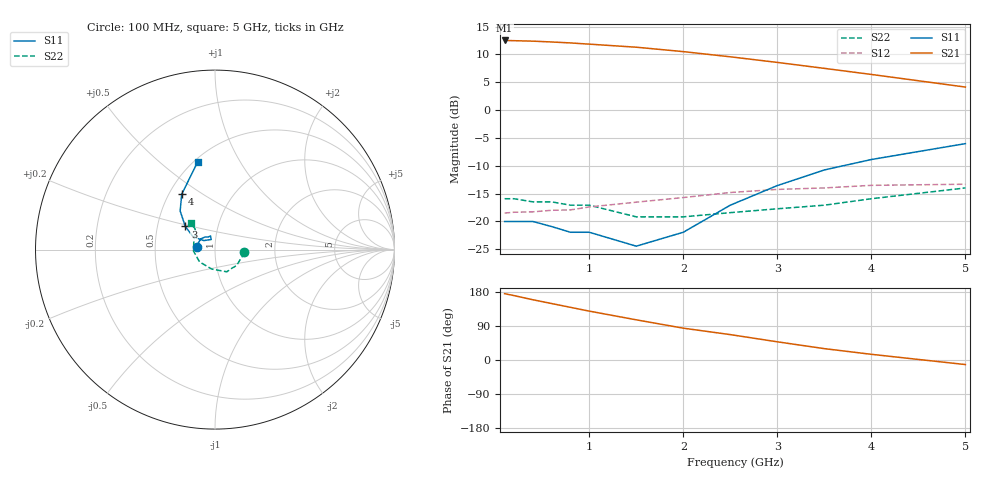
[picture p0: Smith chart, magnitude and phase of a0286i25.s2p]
!  MSA-0286 S AND NOISE PARAMETERS
!  Id=25mA  LAST UPDATED 07-22-92
# ghz s ma r 50
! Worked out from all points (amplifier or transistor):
!   13 points, 100 MHz to 5 GHz, reference 50 ohm
!   highest |S21| = 12.5 dB at 100 MHz (marker M1)
!   |S21| within 3 dB of that: start of sweep to 2.532 GHz
!   unconditionally stable (mu >= 1): start of sweep to end of sweep
!   at 400 MHz: K = 1.20, MAG = 12.6 dB, |S12| = -18.3 dB
!   at 1.5 GHz: K = 1.18, MAG = 11.4 dB, |S12| = -16.5 dB
!   at 5 GHz: K = 1.23, MAG = 5.8 dB, |S12| = -13.3 dB
!   lowest NFmin = 6.00 dB at 100 MHz
!   S11 on the Smith chart (normalised r, x): 100 MHz: 0.82, +0.03; 3 GHz: 0.70, +0.19; 4 GHz: 0.58, +0.41; 5 GHz: 0.52, +0.68
0.1  0.1 171.0  4.22 175.0  0.119 1.0  0.16 -5.0
0.2  0.1 161.0  4.2 170.0  0.121 3.0  0.16 -11.0
0.4  0.1 144.0  4.16 159.0  0.122 6.0  0.15 -24.0
0.6  0.09 129.0  4.09 149.0  0.126 6.0  0.15 -36.0
0.8  0.08 119.0  4.01 139.0  0.127 9.0  0.14 -48.0
1  0.08 108.0  3.91 129.0  0.135 8.0  0.14 -62.0
1.5  0.06 111.0  3.67 106.0  0.149 12.0  0.11 -99.0
2  0.08 141.0  3.35 84.0  0.164 11.0  0.11 -141.0
2.5  0.14 150.0  3.01 67.0  0.182 9.0  0.12 -176.0
3  0.21 142.0  2.68 48.0  0.194 5.0  0.13 155.0
3.5  0.29 132.0  2.37 30.0  0.2 1.0  0.14 140.0
4  0.36 121.0  2.09 15.0  0.211 -3.0  0.16 134.0
5  0.5 101.0  1.61 -12.0  0.216 -12.0  0.2 132.0
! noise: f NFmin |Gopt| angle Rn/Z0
0.1  6  0.09  -2  1.15
0.5  6.3  0.08  -7  1.15
1  6.5  0.08  -20  1.14
2  6.9  0.08  -50  1.12
